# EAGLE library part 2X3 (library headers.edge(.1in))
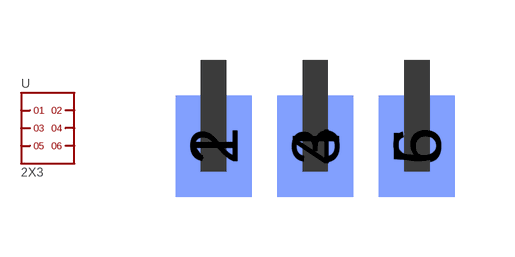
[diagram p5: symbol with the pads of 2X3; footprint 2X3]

Designator prefix -

## 2X3  [2X3]
1  1
2  2
3  3
4  4
5  5
6  6

## Footprint 2X3 (pad centres in mm)
smd 1.905 x 2.54: 1 0,-2.159; 3 2.54,-2.159; 5 5.08,-2.159
smd 1.905 x 2.54 bottom: 2 0,-2.159; 4 2.54,-2.159; 6 5.08,-2.159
